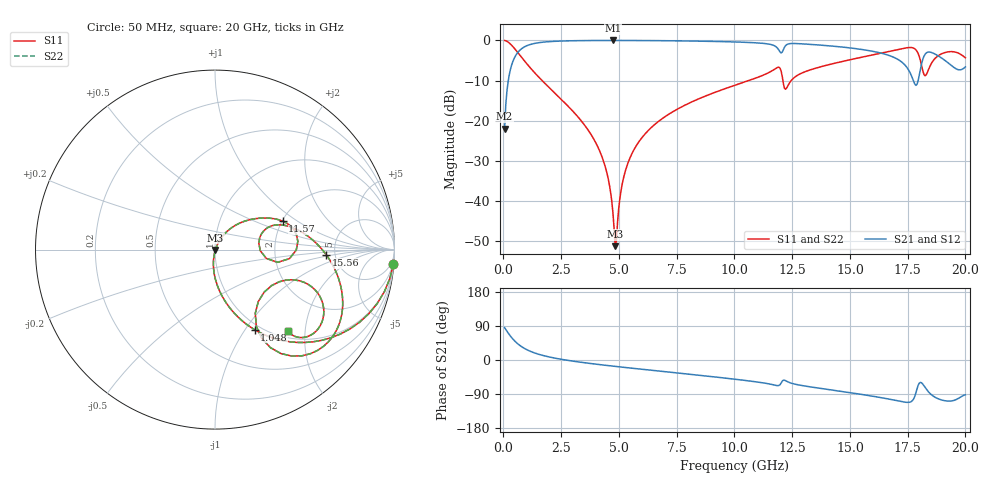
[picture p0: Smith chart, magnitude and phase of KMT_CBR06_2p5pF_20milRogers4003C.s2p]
! Data measured by Modelithics Inc. support@modelithics.com 813-866-6335
! KEMET CBR0603 2.5pF, Pad Width= 0.851mm, Pad Length= 0.64mm, Pad Gap= 0.62mm, 20mil Rogers 4003C substrate Data, January 2022
# hz S ma R 50
! 2 Port Network Data from SP1.SP block
! freq  magS11  angS11  magS21  angS21  magS12  angS12  magS22  angS22
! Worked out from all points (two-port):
!   401 points, 50 MHz to 20 GHz, reference 50 ohm
!   highest |S21| = -0.02 dB at 4.738 GHz (marker M1); lowest = -22.0 dB at 50 MHz (marker M2)
!   |S21| within 3 dB of the highest: 618.7 MHz to 12 GHz (11.38 GHz wide, 180 % of centre); 12.05 GHz to 16.24 GHz (4.19 GHz wide, 29.6 % of centre)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
!   lowest |S11| = -51.2 dB at 4.838 GHz (marker M3), VSWR 1.01, Z = 50.2 - j0.173 ohm
!   |S11| at or under -10 dB: 1.673 GHz to 10.62 GHz (8.942 GHz wide, 146 % of centre); 12.1 GHz to 12.46 GHz (360.9 MHz wide, 2.94 % of centre)
!   |S22| runs from -51.2 to 0.0 dB; largest |S21 - S12| = 0
!   S11 on the Smith chart (normalised r, x): 50 MHz: 1, -24; 1.048 GHz: 0.93, -1.10; 11.57 GHz: 2.01, +0.77; 15.56 GHz: 4.24, -0.42; 20 GHz: 1.13, -1.62
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5e7  0.9968 -4.7  0.07936 85.3  0.07936 85.3  0.9968 -4.7
3.99125e8  0.842 -34.0  0.5384 56.0  0.5384 56.0  0.842 -34.0
1.0475e9  0.4971 -63.7  0.8663 26.1  0.8663 26.1  0.4971 -63.7
3.391625e9  0.09786 -95.0  0.9929 -6.3  0.9929 -6.3  0.09786 -95.0
4.33925e9  0.03103 -98.9  0.9969 -13.4  0.9969 -13.4  0.03103 -98.9
4.73825e9  0.007262 -85.8  0.9973 -16.2  0.9973 -16.2  0.007262 -85.8
4.838e9  0.002755 -38.6  0.9973 -16.9  0.9973 -16.9  0.002755 -38.6
5.4365e9  0.03229 64.3  0.9966 -20.8  0.9966 -20.8  0.03229 64.3
6.73325e9  0.09919 59.0  0.9917 -29.2  0.9917 -29.2  0.09919 59.0
1.0025e10  0.2768 38.2  0.9555 -50.7  0.9555 -50.7  0.2768 38.2
1.157112e10  0.409 22.9  0.8894 -63.9  0.8894 -63.9  0.409 22.9
1.192025e10  0.4638 5.7  0.7606 -67.3  0.7606 -67.3  0.4638 5.7
1.226938e10  0.2579 15.0  0.8864 -56.3  0.8864 -56.3  0.2579 15.0
1.336662e10  0.4372 16.9  0.888 -71.7  0.888 -71.7  0.4372 16.9
1.556112e10  0.6216 -2.8  0.767 -91.3  0.767 -91.3  0.6216 -2.8
1.670825e10  0.7299 -16.3  0.647 -103.4  0.647 -103.4  0.7299 -16.3
1.745638e10  0.8085 -31.6  0.4653 -111.8  0.4653 -111.8  0.8085 -31.6
1.785538e10  0.7641 -50.8  0.2756 -87.2  0.2756 -87.2  0.7641 -50.8
1.815462e10  0.4203 -57.7  0.5803 -63.6  0.5803 -63.6  0.4203 -57.7
1.845388e10  0.4687 -21.0  0.7155 -87.6  0.7155 -87.6  0.4687 -21.0
1.895262e10  0.6772 -27.2  0.6073 -105.2  0.6073 -105.2  0.6772 -27.2
2e10  0.6073 -48.1  0.4674 -91.7  0.4674 -91.7  0.6073 -48.1
